FUNCTION_BLOCK FB_DO_IED_LD1_LEDGGIO5_SPCSO1 EXTENDS FB_AcsiCommonControllableDataClass
VAR_INPUT
	stVal: FB_AcsiBATypeBOOLEAN := (fc:=ACSI_FC_ST, TrgOp:=ACSI_TrgOp_dchg, bLinkResult:=THIS^.AddDataToContainer(ipData:=stVal));
	q: FB_AcsiDATypeQuality := (fc:=ACSI_FC_ST, TrgOp:=ACSI_TrgOp_qchg, bLinkResult:=THIS^.AddDataToContainer(ipData:=q));
	t: FB_AcsiDATypeTimeStamp := (fc:=ACSI_FC_ST, bLinkResult:=THIS^.AddDataToContainer(ipData:=t));
	stSeld: FB_AcsiBATypeBOOLEAN := (fc:=ACSI_FC_ST, TrgOp:=ACSI_TrgOp_dchg, bLinkResult:=THIS^.AddDataToContainer(ipData:=stSeld));
	ctlModel: FB_AcsiDATypeCtlModels := (fc:=ACSI_FC_CF, TrgOp:=ACSI_TrgOp_dchg, eValue:=E_AcsiCtlModels.SBOWithEnhancedSecurity, bLinkResult:=THIS^.AddDataToContainer(ipData:=ctlModel));
	sboTimeout: FB_AcsiBATypeINT32U := (fc:=ACSI_FC_CF, TrgOp:=ACSI_TrgOp_dchg, nValue:=30000, bLinkResult:=THIS^.AddDataToContainer(ipData:=sboTimeout));
	sboClass: FB_AcsiDATypeSboClasses := (fc:=ACSI_FC_CF, TrgOp:=ACSI_TrgOp_dchg, eValue:=E_AcsiSboClasses.OperateOnce, bLinkResult:=THIS^.AddDataToContainer(ipData:=sboClass));
	operTimeout: FB_AcsiBATypeINT32U := (fc:=ACSI_FC_CF, TrgOp:=ACSI_TrgOp_dchg, nValue:=30000, bLinkResult:=THIS^.AddDataToContainer(ipData:=operTimeout));
	Oper: FB_AcsiCDC_Oper_BOOLEAN := (fc:=ACSI_FC_CO, bLinkResult:=THIS^.AddDataToContainer(ipData:=Oper));
	SBOw: FB_AcsiCDC_SBOw_BOOLEAN := (fc:=ACSI_FC_CO, bLinkResult:=THIS^.AddDataToContainer(ipData:=SBOw));
	Cancel: FB_AcsiCDC_Cancel_BOOLEAN := (fc:=ACSI_FC_CO, bLinkResult:=THIS^.AddDataToContainer(ipData:=Cancel));
	
	fbControl: FB_SboControl := (ipCtrl:=THIS^.AddServerJob(ipEvent:=fbControl, ipCompletion:=fbControl), eType:=E_AcsiCDCType.SPC, ipBehVal:=fbIED.IEDLD1.LEDGGIO5.Beh.stVal);
END_VAR
VAR
END_VAR

END_FUNCTION_BLOCK
